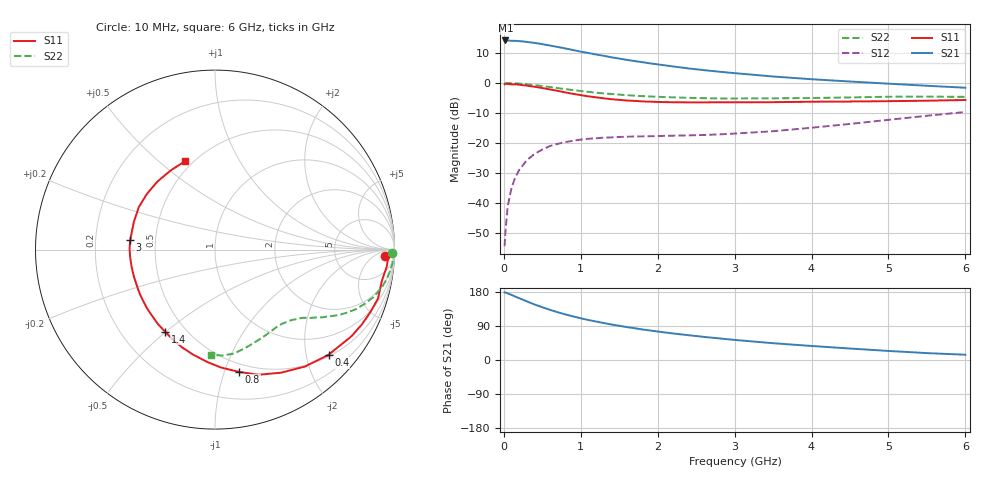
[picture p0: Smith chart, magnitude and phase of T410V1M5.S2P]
! Infineon Technologies  Discrete & RF Semiconductors
! BFR182T
! Si NPN RF Bipolar Junction Transistor in SC75
! VCE = 10 V  IC = 1.5 mA
! Common Emitter S-Parameters:  October  1999
# GHz  S  MA  R  50
!  f  S11  S21  S12  S22
! GHz  MAG  ANG  MAG  ANG  MAG  ANG  MAG  ANG
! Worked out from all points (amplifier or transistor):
!   36 points, 10 MHz to 6 GHz, reference 50 ohm
!   highest |S21| = 14.2 dB at 20 MHz (marker M1)
!   |S21| within 3 dB of that: start of sweep to 863 MHz
!   unconditionally stable (mu >= 1): 2.264 GHz to 4.545 GHz
!   at 250 MHz: K = 0.11, MSG = 20.6 dB, |S12| = -27.3 dB
!   at 1.4 GHz: K = 0.67, MSG = 13.3 dB, |S12| = -18.2 dB
!   at 6 GHz: K = 0.83, MSG = 4.0 dB, |S12| = -9.7 dB
!   S11 on the Smith chart (normalised r, x): 10 MHz: 26, -18; 400 MHz: 0.54, -2.45; 800 MHz: 0.43, -1.12; 1.4 GHz: 0.39, -0.50; 3 GHz: 0.36, +0.05; 6 GHz: 0.45, +0.61
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0.01  0.949 -2.1  5.071 178.4  0.0019 76.8  0.9886 -1.2
0.02  0.9691 -0.9  5.106 178.5  0.0032 86.6  0.9957 -0.9
0.05  0.9615 -5.7  5.095 175.6  0.0088 89.3  0.9934 -2.3
0.1  0.9459 -10.6  5.036 171.8  0.0178 85.5  0.9917 -4.5
0.15  0.9484 -16.7  5.034 167.3  0.0268 80.3  0.983 -6.8
0.25  0.9185 -27.0  4.913 158.8  0.043 74.4  0.9636 -11.0
0.4  0.8624 -42.8  4.651 146.5  0.0656 66.1  0.9203 -16.8
0.5  0.8222 -52.4  4.43 139.3  0.0777 61.0  0.8871 -19.9
0.6  0.7782 -61.8  4.202 132.3  0.0887 56.9  0.8538 -22.8
0.8  0.6948 -78.8  3.76 120.3  0.1035 49.8  0.7883 -27.3
0.9  0.6578 -87.1  3.532 115.0  0.1084 47.0  0.7585 -29.1
1.1  0.5978 -101.7  3.155 105.4  0.1173 42.7  0.7098 -32.1
1.4  0.5349 -121.4  2.672 93.7  0.1237 38.6  0.6542 -35.6
1.6  0.5089 -133.5  2.42 86.8  0.127 37.3  0.6249 -37.4
1.8  0.4921 -144.1  2.222 80.6  0.1287 37.2  0.6021 -39.7
2.2  0.4762 -161.1  1.883 70.0  0.1321 38.3  0.5748 -43.5
2.6  0.4747 -175.1  1.634 61.0  0.1357 41.4  0.5564 -48.2
3  0.4754 173.7  1.456 53.0  0.1431 45.1  0.5512 -52.5
3.5  0.4776 161.3  1.28 44.3  0.1567 50.2  0.5538 -59.1
4.5  0.4901 140.8  1.056 30.3  0.2074 57.2  0.5733 -72.7
5.5  0.5054 119.3  0.897 18.2  0.2835 57.7  0.5918 -86.1
6  0.5198 108.9  0.832 13.9  0.3277 55.4  0.586 -92.3
